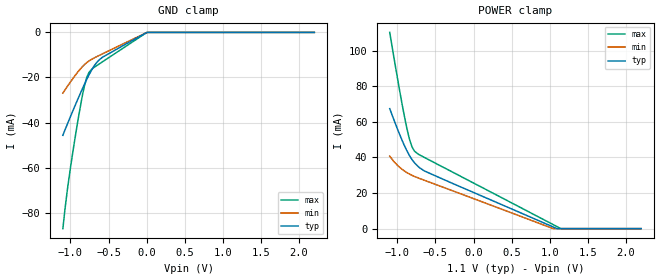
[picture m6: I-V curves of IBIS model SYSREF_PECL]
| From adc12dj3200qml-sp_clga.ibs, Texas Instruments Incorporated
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[Model]   SYSREF_PECL
Model_type   Input
Vinl = 0.33   | Vinl & Vinh are referred to a 1.1V supply, and are an IBIS required field.
Vinh = 0.77   | However, please note that this is a differential input.
|   typ   min   max
C_comp   1.02p   0.95p   1.09p
[Voltage Range]   1.1   1.05   1.15
[Temperature Range]   25   125   -40
[Power Clamp Reference]   1.1   1.05   1.15
[GND Clamp Reference]   0   0   0
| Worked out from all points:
|   GND clamp passes 1 mA (typ) near -0.05 V on its own axis
[GND Clamp]
|   Voltage   I(typ)   I(min)   I(max)
-1.1V     -45.65mA   -26.92mA   -87.06mA
-1.037V   -40.39mA   -23.78mA   -68.93mA
-1.001V   -37.42mA   -22.01mA   -60.22mA
-911.9mV  -30.28mA   -17.92mA   -41.03mA
-852.5mV  -25.69mA   -15.53mA   -29.59mA
-816.2mV  -23mA      -14.28mA   -23.7mA
-783.2mV  -20.65mA   -13.32mA   -19.72mA
-753.5mV  -18.64mA   -12.6mA    -17.58mA
-713.9mV  -16.2mA    -11.79mA   -16.14mA
-581.9mV  -11.07mA   -9.533mA   -13.08mA
2.2mV     -32.23uA   -38.49uA   -12.4uA
2.2V      0A         0A         0A
[POWER Clamp]
|   Voltage   I(typ)   I(min)   I(max)
-1.1V     67.39mA    40.71mA    110.2mA
-984.5mV  54.46mA    35mA       81.08mA
-918.5mV  47.73mA    32.74mA    65.57mA
-875.6mV  43.82mA    31.52mA    56.52mA
-839.3mV  40.94mA    30.62mA    50.12mA
-809.6mV  38.94mA    29.99mA    46.27mA
-776.6mV  37.08mA    29.35mA    43.7mA
-730.4mV  35.01mA    28.56mA    41.99mA
-644.6mV  32.39mA    27.17mA    39.99mA
1.045V    950.2uA    6.969uA    2.287mA
1.144V    0A         0A         72.62uA
2.2V      0A         0A         0A
